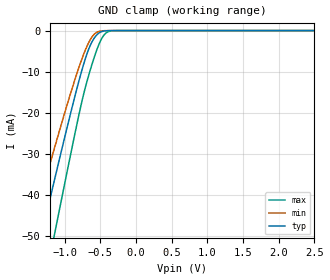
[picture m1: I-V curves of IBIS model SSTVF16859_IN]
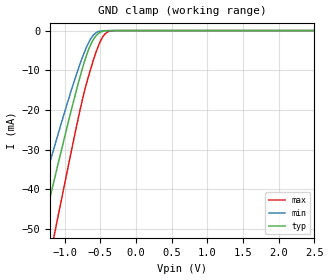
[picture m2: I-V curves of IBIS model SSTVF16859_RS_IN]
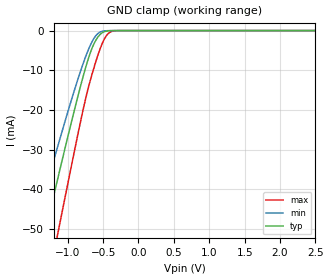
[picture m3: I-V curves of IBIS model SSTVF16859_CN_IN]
| TEXAS INSTRUMENTS INCORPORATED
| Standard Linear and Logic Group
| IBIS Model of SN74SSTVF16859DGG
| 13-BIT to 26-BIT Registered Buffer w/SSTL2 Input and Outputs
| This file contains package information for the following:
|  TSSOP 64-pin (DGG) package as [Component] SSTVF16859_DGG
| This device can be powered at the following Vccs:
|  2.5 volt Vcc
| This file provides unique models under the [Model Selector] for each Vcc.
| For operation at a specific Vcc, select the appropriate model after each
| [Model Selector] keyword.
[IBIS Ver]   3.2
[Comment char]  |_char
[File Name]   sn74sstvf16859dgg.ibs
[File Rev]   1.1 | X
[Date]   February 10, 2003
[Source]   Data created from TI-SPICE simulations at TI-SLL.
[Notes]   The following is an IBIS list for the SSTVF16859_DGG.
   Please contact sllibis@ti.com with questions and
   comments concerning SLL IBIS models.
   -As there is no power clamp diode in the Input model,
   we removed the Power Clamp table data from the Input model
   -For differential type input Vinl and Vinh should be
   set as optional, but since IBIS pursers give error, we
   set dummy values of Vinh and Vinl
   -An IBIS model does not adequately simulate the dynamic
   behavior of the multi-stage output driver in the SN74SSTVF16859
   device. TI recommends that customers do NOT use the IBIS model.
   For more accurate simulation results, please use the HSPICE
   model if you can.
[Disclaimer] Property of Texas Instruments Incorporated.  Unauthorized
   reproduction and/or distribution is strictly prohibited.
   This product is protected under copyright law.
   Created  2003, (C) Copyright  2003, Texas Instruments
   Incorporated, All Rights Reserved
   UNLESS THERE IS A SIGNED, WRITTEN AGREEMENT TO THE
   CONTRARY, TEXAS INSTRUMENTS (TI) IS PROVIDING THE IBIS
   MODELS  AND WITHOUT ANY WARRANTY, EXPRESSED OR
   IMPLIED.  TI assumes no liability for:
   1) the accuracy of the IBIS models provided to your
   company;
   2) the proper functioning of these IBIS Models in your
   design or for any resulting applications; or
   3) infringement of patents, copyrights or intellectual
   property rights resulting from your use of these IBIS
   models.
   TI provides IBIS Models as a service to our customers.
   You and your company shall not distribute, sell or give
   these models to anyone else without prior written
   permission from TI.
   TI reserves the right to make changes to our products or
   to discontinue any semiconductor product or service
   without notice, and advises our customers to obtain the
   latest version of relevant information to verify, before
   placing orders, that the information being relied on is
   current.
   Please be aware that your receipt and use of the IBIS
   information provided shall serve as acceptance of these
   terms and conditions.  If you do not accept these terms,
   you should return or destroy the IBIS models and any
   other accompanying information immediately.
| Component SSTVF16859_DGG 64-pin TSSOP
[Component]   SSTVF16859_DGG
[Manufacturer]   Texas Instruments, Inc.
[Package]
|   typ   min   max
R_pkg   6.000e-02   4.900e-02   7.800e-02
L_pkg   3.977e-09   2.954e-09   5.572e-09
C_pkg   5.910e-13   3.330e-13   1.005e-12
[Pin]   signal_name   model_name   R_pin   L_pin   C_pin
1   Q13A   SSTVF16859_OUT   6.300e-02   5.570e-09   9.070e-13
2   Q12A   SSTVF16859_OUT   5.700e-02   5.101e-09   9.840e-13
3   Q11A   SSTVF16859_OUT   6.200e-02   4.902e-09   9.050e-13
4   Q10A   SSTVF16859_OUT   6.400e-02   4.735e-09   8.140e-13
5   Q9A   SSTVF16859_OUT   6.800e-02   4.600e-09   7.240e-13
6   VDDQ   POWER   7.300e-02   4.461e-09   6.320e-13
7   GND   GND   7.400e-02   4.301e-09   5.760e-13
8   Q8A   SSTVF16859_OUT   6.900e-02   3.957e-09   5.660e-13
9   Q7A   SSTVF16859_OUT   5.100e-02   3.670e-09   5.180e-13
10   Q6A   SSTVF16859_OUT   5.100e-02   3.495e-09   4.480e-13
11   Q5A   SSTVF16859_OUT   5.200e-02   3.364e-09   4.270e-13
12   Q4A   SSTVF16859_OUT   5.100e-02   3.262e-09   4.150e-13
13   Q3A   SSTVF16859_OUT   5.300e-02   3.152e-09   3.870e-13
14   Q2A   SSTVF16859_OUT   5.300e-02   3.073e-09   3.680e-13
15   GND   GND   5.400e-02   3.010e-09   3.530e-13
16   Q1A   SSTVF16859_OUT   5.400e-02   2.956e-09   3.350e-13
17   Q13B   SSTVF16859_OUT   5.400e-02   2.954e-09   3.350e-13
18   VDDQ   POWER   5.400e-02   3.010e-09   3.530e-13
19   Q12B   SSTVF16859_OUT   5.300e-02   3.069e-09   3.680e-13
20   Q11B   SSTVF16859_OUT   5.300e-02   3.149e-09   3.850e-13
21   Q10B   SSTVF16859_OUT   5.100e-02   3.240e-09   4.060e-13
22   Q9B   SSTVF16859_OUT   5.200e-02   3.360e-09   4.260e-13
23   Q8B   SSTVF16859_OUT   5.000e-02   3.485e-09   4.470e-13
24   Q7B   SSTVF16859_OUT   5.000e-02   3.661e-09   5.260e-13
25   Q6B   SSTVF16859_OUT   6.900e-02   3.949e-09   5.940e-13
26   GND   GND   7.500e-02   4.292e-09   6.070e-13
27   VDDQ   POWER   7.200e-02   4.443e-09   6.570e-13
28   Q5B   SSTVF16859_OUT   6.900e-02   4.588e-09   7.470e-13
29   Q4B   SSTVF16859_OUT   6.400e-02   4.723e-09   8.370e-13
30   Q3B   SSTVF16859_OUT   6.200e-02   4.892e-09   9.270e-13
31   Q2B   SSTVF16859_OUT   5.700e-02   5.093e-09   9.990e-13
32   Q1B   SSTVF16859_OUT   6.300e-02   5.572e-09   9.070e-13
33   VDDQ   POWER   5.600e-02   5.516e-09   9.110e-13
34   GND   GND   6.000e-02   5.173e-09   9.900e-13
35   D1   SSTVF16859_IN   6.200e-02   4.898e-09   9.000e-13
36   D2   SSTVF16859_IN   6.400e-02   4.723e-09   8.190e-13
37   VCC   POWER   7.100e-02   4.594e-09   7.350e-13
38   VDDQ   POWER   7.500e-02   4.456e-09   6.480e-13
39   GND   GND   7.700e-02   4.301e-09   5.920e-13
40   D3   SSTVF16859_IN   7.300e-02   3.961e-09   5.780e-13
41   D4   SSTVF16859_IN   5.000e-02   3.661e-09   5.210e-13
42   D5   SSTVF16859_IN   5.000e-02   3.487e-09   4.460e-13
43   GND   GND   5.100e-02   3.345e-09   4.250e-13
44   D6   SSTVF16859_IN   5.200e-02   3.224e-09   4.040e-13
45   VREF   SSTVF16859_VR_IN   5.300e-02   3.126e-09   3.790e-13
46   VCC   POWER   5.300e-02   3.070e-09   3.630e-13
47   VDDQ   POWER   5.400e-02   3.011e-09   3.500e-13
48   CLK   SSTVF16859_CP_IN   5.400e-02   2.956e-09   3.330e-13
49   CLK_   SSTVF16859_CN_IN   5.400e-02   2.957e-09   3.330e-13
50   GND   GND   5.300e-02   3.009e-09   3.510e-13
51   RESET_   SSTVF16859_RS_IN   5.300e-02   3.073e-09   3.660e-13
52   D7   SSTVF16859_IN   5.300e-02   3.152e-09   3.850e-13
53   D8   SSTVF16859_IN   5.100e-02   3.256e-09   4.140e-13
54   GND   GND   5.100e-02   3.375e-09   4.300e-13
55   D9   SSTVF16859_IN   5.100e-02   3.538e-09   4.530e-13
56   D10   SSTVF16859_IN   4.900e-02   3.721e-09   5.380e-13
57   D11   SSTVF16859_IN   7.500e-02   4.067e-09   5.950e-13
58   GND   GND   7.800e-02   4.315e-09   5.970e-13
59   VDDQ   POWER   7.600e-02   4.468e-09   6.560e-13
60   VCC   POWER   7.000e-02   4.603e-09   7.460e-13
61   D12   SSTVF16859_IN   6.500e-02   4.739e-09   8.320e-13
62   D13   SSTVF16859_IN   6.300e-02   4.915e-09   9.140e-13
63   GND   GND   6.100e-02   5.191e-09   1.005e-12
64   VDDQ   POWER   5.900e-02   5.541e-09   9.230e-13
| Models and submodels in the file (6): SSTVF16859_IN (Input), SSTVF16859_RS_IN (Input), SSTVF16859_CN_IN (Input), SSTVF16859_CP_IN (Input), SSTVF16859_VR_IN (Input), SSTVF16859_OUT (Output)
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| NOTE:  The [Diff Pin] section is commented out because the ibischk3 program
|   currently flags it as an Error when it shouldn't
| [Diff Pin]  inv_pin   vdiff   tdelay_typ
|48   49   0.180   0
|35   45   0.310   0
|36   45   0.310   0
|40   45   0.310   0
|41   45   0.310   0
|42   45   0.310   0
|44   45   0.310   0
|52   45   0.310   0
|53   45   0.310   0
|55   45   0.310   0
|56   45   0.310   0
|57   45   0.310   0
|61   45   0.310   0
|62   45   0.310   0
[Model]   SSTVF16859_IN
Model_type  Input
Vinh=0.97
Vinl=1.53
| variable   typ   min   max
|C_comp   1.77pF   1.41pF   2.16pF
C_comp   3.04pF   2.94pF   3.14pF
|Note: The above cap values are based on Back-Annotation by Roman Pacheco
[Temperature Range]   40   85   0
| Ambient temperature   25   70   0
[Voltage range]   2.5   2.5   2.5
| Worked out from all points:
|   GND clamp passes 1 mA (typ) near -0.55 V on its own axis
[GND Clamp]
| SSTVF16859_IN
|   Voltage   I(typ)   I(min)   I(max)
-2.5V     -138.9mA   -116.4mA   -166.4mA
-1.49V    -62.29mA   -50.36mA   -79.78mA
-1.44V    -58.54mA   -47.18mA   -75.45mA
-1.305V   -48.45mA   -38.68mA   -63.77mA
-1.14V    -36.26mA   -28.51mA   -49.49mA
-1.1V     -33.34mA   -26.09mA   -46.04mA
-750mV    -9.216mA   -6.589mA   -16.74mA
-655mV    -4.225mA   -2.699mA   -10.49mA
-555mV    -1.172mA   -492.4uA   -5.026mA
-445mV    -108.7uA   -34uA      -1.041mA
-325mV    -3.339uA   -1.231uA   -42.72uA
2.5V      313.9pA    204.1pA    3.455nA
[Model]   SSTVF16859_RS_IN
Model_type  Input
Vinl=0.7
Vinh=1.7
| variable   typ   min   max
|C_comp   1.83pF   1.46pF   2.23pF
C_comp   3.04pF   2.62pF   3.46pF
|Note: The above cap values are based on Back-Annotation by Roman Pacheco
[Temperature Range]   40   85   0
| Ambient temperature   25   70   0
[Voltage range]   2.5   2.3   2.7
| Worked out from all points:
|   GND clamp passes 1 mA (typ) near -0.54 V on its own axis
[GND Clamp]
| SSTVF16859_RS_IN
|   Voltage   I(typ)   I(min)   I(max)
-2.5V     -142.5mA   -119mA     -171.5mA
-1.49V    -63.97mA   -51.46mA   -82.34mA
-1.44V    -60.12mA   -48.21mA   -77.9mA
-1.305V   -49.78mA   -39.54mA   -65.87mA
-1.14V    -37.28mA   -29.15mA   -51.17mA
-910mV    -20.37mA   -15.32mA   -30.82mA
-745mV    -9.239mA   -6.51mA    -17.05mA
-650mV    -4.192mA   -2.605mA   -10.64mA
-550mV    -1.134mA   -458.4uA   -5.008mA
-445mV    -115.2uA   -35.68uA   -1.098mA
-325mV    -3.541uA   -1.298uA   -45.32uA
2.5V      338.1pA    223.4pA    3.669nA
[Model]   SSTVF16859_CN_IN
Model_type  Input
Vinh=0.97
Vinl=1.53
| variable   typ   min   max
|C_comp   1.89pF   1.51pF   2.30pF
C_comp   3.03pF   2.98pF   3.08pF
|Note: The above cap values are based on Back-Annotation by Roman Pacheco
[Temperature Range]   40   85   0
| Ambient temperature   25   70   0
[Voltage range]   2.5   2.3   2.7
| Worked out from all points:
|   GND clamp passes 1 mA (typ) near -0.54 V on its own axis
[GND Clamp]
| SSTVF16859_CN_IN
|   Voltage   I(typ)   I(min)   I(max)
-2.5V     -142.5mA   -119mA     -171.5mA
-1.49V    -63.97mA   -51.46mA   -82.34mA
-1.44V    -60.12mA   -48.21mA   -77.9mA
-1.305V   -49.78mA   -39.54mA   -65.87mA
-1.14V    -37.28mA   -29.15mA   -51.17mA
-910mV    -20.37mA   -15.32mA   -30.82mA
-745mV    -9.239mA   -6.51mA    -17.05mA
-650mV    -4.192mA   -2.605mA   -10.64mA
-550mV    -1.134mA   -458.4uA   -5.008mA
-445mV    -115.2uA   -35.68uA   -1.098mA
-325mV    -3.541uA   -1.298uA   -45.32uA
2.5V      338.1pA    223.4pA    3.669nA
